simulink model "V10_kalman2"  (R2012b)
settings: Solver=FixedStepDiscrete  StartTime=0.0  StopTime=20  FixedStep=0.1  RelTol=1e-3
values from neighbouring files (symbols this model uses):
  Ts = 0.1    [V2_4_tdomain.m]    (also in V2_6_UTFDiskretizierung.m; V2_7_multiZ.m; DBDisk.m = 0.02; DBDisk2.m = 0.02)
undefined symbols (not defined in the file or in its folder): ro, sigma, xo
libraries: simulink x1

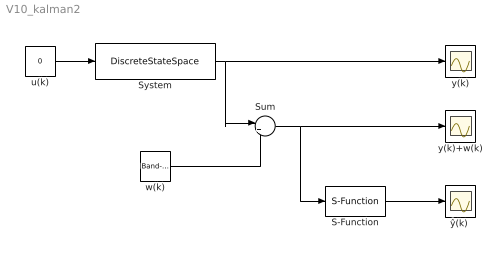
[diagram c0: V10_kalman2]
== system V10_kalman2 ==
  S-Function : S-Function  FunctionName=kalman2  Parameters=sigma,Ts,xo,ro  SFunctionDeploymentMode=off  EnableBusSupport=off
  Sum : Sum  Inputs=|++
  System : DiscreteStateSpace  D=0  X0=5  SampleTime=0.1
  u(k) : Constant  Value=0
  w(k) : simulink/Sources/Band-Limited White Noise  Cov=[0.1]  Ts=0.1  seed=[23341]
  y(k) : Scope
  y(k)+w(k) : Scope
  "ŷ(k) " : Scope
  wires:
  System/1 -> y(k)/1, Sum/1
  u(k)/1 -> System/1
  w(k)/1 -> Sum/2
  Sum/1 -> y(k)+w(k)/1, S-Function/1
  S-Function/1 -> "ŷ(k) "/1
